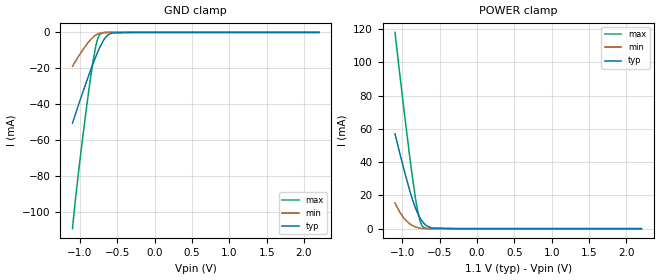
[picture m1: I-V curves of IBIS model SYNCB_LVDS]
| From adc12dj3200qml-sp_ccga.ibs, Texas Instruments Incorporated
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|   Model SYNCB_LVDS
[Model]   SYNCB_LVDS
Model_type   Input
Vinl = 0.33   | Vinl & Vinh are referred to a 1.1V supply, and are an IBIS required field.
Vinh = 0.77   | However, please note that this is a differential input.
|   typ   min   max
C_comp   1.32pF   1.25pF   1.43pF
[Voltage Range]   1.1   1.05   1.15
[Temperature Range]   25   125   -40
[Power Clamp Reference]   1.1   1.05   1.15
[GND Clamp Reference]   0   0   0
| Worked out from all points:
|   GND clamp passes 1 mA (typ) near -0.61 V on its own axis
|   POWER clamp passes 1 mA (typ) near -0.64 V on its own axis
[GND Clamp]
|   Voltage   I(typ)   I(min)   I(max)
-1.1V     -50.43mA   -18.81mA   -109.1mA
-1.064V   -45.8mA    -16.33mA   -94.16mA
-1.018V   -40.05mA   -13.26mA   -77.06mA
-905.3mV  -26.57mA   -6.434mA   -39.65mA
-852.5mV  -20.52mA   -3.788mA   -23.7mA
-819.5mV  -16.88mA   -2.449mA   -14.81mA
-789.8mV  -13.74mA   -1.511mA   -8.093mA
-760.1mV  -10.76mA   -849.9uA   -3.352mA
-730.4mV  -8.01mA    -439.5uA   -994.1uA
-664.4mV  -3.127mA   -84.19uA   -36.95uA
-568.7mV  -300.4uA   -6.635uA   -535.4nA
2.2V      0A         0A         0A
[POWER Clamp]
|   Voltage   I(typ)   I(min)   I(max)
-1.1V     57.02mA    15.46mA    117.9mA
-981.2mV  35.79mA    6.35mA     72.05mA
-908.6mV  23.89mA    3.168mA    45.41mA
-842.6mV  14.49mA    1.353mA    23.37mA
-809.6mV  10.6mA     769.5uA    14mA
-786.5mV  8.295mA    485.8uA    8.602mA
-763.4mV  6.343mA    292.1uA    4.548mA
-743.6mV  4.94mA     183uA      2.281mA
-710.6mV  3.086mA    80.3uA     552.5uA
-614.9mV  411.5uA    6.508uA    5.182uA
-275mV    32.08nA    2.095nA    115.5nA
2.2V      0A         0A         0A
